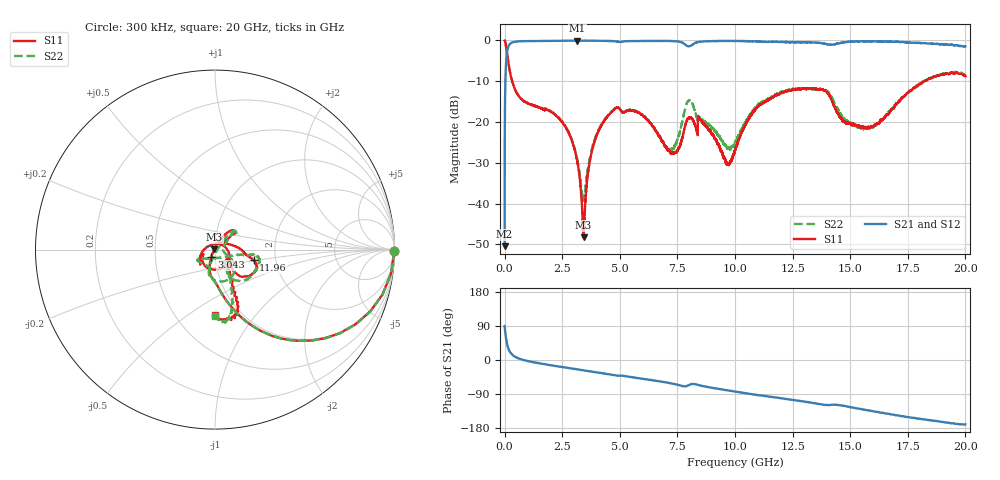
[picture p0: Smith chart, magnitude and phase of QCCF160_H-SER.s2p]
!{QCCF160}
!Johanson Technology Inc.
!www.johansontechnology.com
!Test Board Conditions:
!Substrate Type  RO4350B
!Substrate Thickness  10 mil
!Substrate Dk  3.66
!TL Type: GCPW
!TL Trace Width  21 mil
!TL Gap  20 mil
!Electrode orientation  Horizontal
!DUT TOPOLOGY	SERIES
!Mounting Pad LxW  16x21 mil
! Created Sat Jan  9 18:20:16 2021
# hz S ma R 50
! 2 Port Network Data from SP1.SP block
! freq  magS11  angS11  magS21  angS21  magS12  angS12  magS22  angS22
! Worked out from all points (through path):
!   20001 points, 300 kHz to 20 GHz, reference 50 ohm
!   highest |S21| = -0.04 dB at 3.156 GHz (marker M1); lowest = -50.5 dB at 300 kHz (marker M2)
!   group delay of S21, straight-line fit = 24.8 ps
!   lowest |S11| = -48.3 dB at 3.426 GHz (marker M3), VSWR 1.01, Z = 49.7 + j0.175 ohm
!   |S11| at or under -10 dB: 328.5 MHz to 18.21 GHz (17.88 GHz wide, 193 % of centre); 18.20895 GHz to 18.20959 GHz (633.7 kHz wide, 0.00348 % of centre)
!   |S22| runs from -39.2 to 0.0 dB; largest |S21 - S12| = 0.014
!   S11 on the Smith chart (normalised r, x): 300 kHz: open; 3.043 GHz: 0.96, -0.08; 11.96 GHz: 1.53, -0.19; 20 GHz: 0.77, -0.64
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300000  0.9983 -0.5  0.003001 89.4  0.003005 88.7  0.9987 -0.5
1.043e8  0.6951 -47.0  0.7138 42.8  0.7147 42.7  0.6961 -46.9
2.173e8  0.4328 -66.7  0.8982 22.6  0.8973 22.7  0.4318 -66.9
9.003e8  0.1754 -90.5  0.9815 -1.2  0.9811 -1.3  0.1763 -91.4
2.3053e9  0.1143 -105.5  0.9888 -16.7  0.9892 -16.7  0.1157 -106.5
3.0433e9  0.04572 -117.1  0.9939 -23.6  0.9947 -23.7  0.04644 -102.9
3.1563e9  0.03267 -120.5  0.9959 -24.7  0.9943 -24.8  0.03383 -99.1
3.3343e9  0.01189 -134.5  0.9948 -26.4  0.9948 -26.4  0.01526 -72.6
3.4263e9  0.00384 152.7  0.9942 -27.3  0.9952 -27.3  0.01099 -25.0
3.8183e9  0.0481 65.2  0.9928 -31.0  0.9938 -31.0  0.05016 44.4
4.5613e9  0.1251 52.8  0.9842 -38.0  0.9848 -38.0  0.1266 47.7
6.6673e9  0.07007 40.2  0.9873 -55.8  0.9873 -55.8  0.06931 31.6
7.2773e9  0.04248 48.5  0.9827 -62.3  0.9834 -62.3  0.04712 -5.7
8.0253e9  0.112 -86.1  0.8495 -65.5  0.8504 -65.5  0.1836 -74.0
9.6723e9  0.03164 113.6  0.9863 -80.0  0.9846 -80.0  0.04762 -96.7
1.00003e10  0.04545 50.3  0.9866 -83.2  0.9843 -83.3  0.05646 -51.5
1.08533e10  0.1388 1.8  0.9783 -91.3  0.976 -91.2  0.1459 -11.4
1.19563e10  0.223 -15.6  0.9591 -100.6  0.9578 -100.6  0.2283 -8.6
1.33343e10  0.2547 -25.7  0.943 -112.8  0.9441 -112.9  0.2546 -22.9
1.53823e10  0.08956 -31.8  0.9702 -128.7  0.971 -128.6  0.08722 -51.6
1.66673e10  0.1257 -54.3  0.962 -142.1  0.9656 -142.4  0.1319 -60.1
2e10  0.363 -89.6  0.8456 -170.0  0.842 -169.9  0.3702 -89.9
